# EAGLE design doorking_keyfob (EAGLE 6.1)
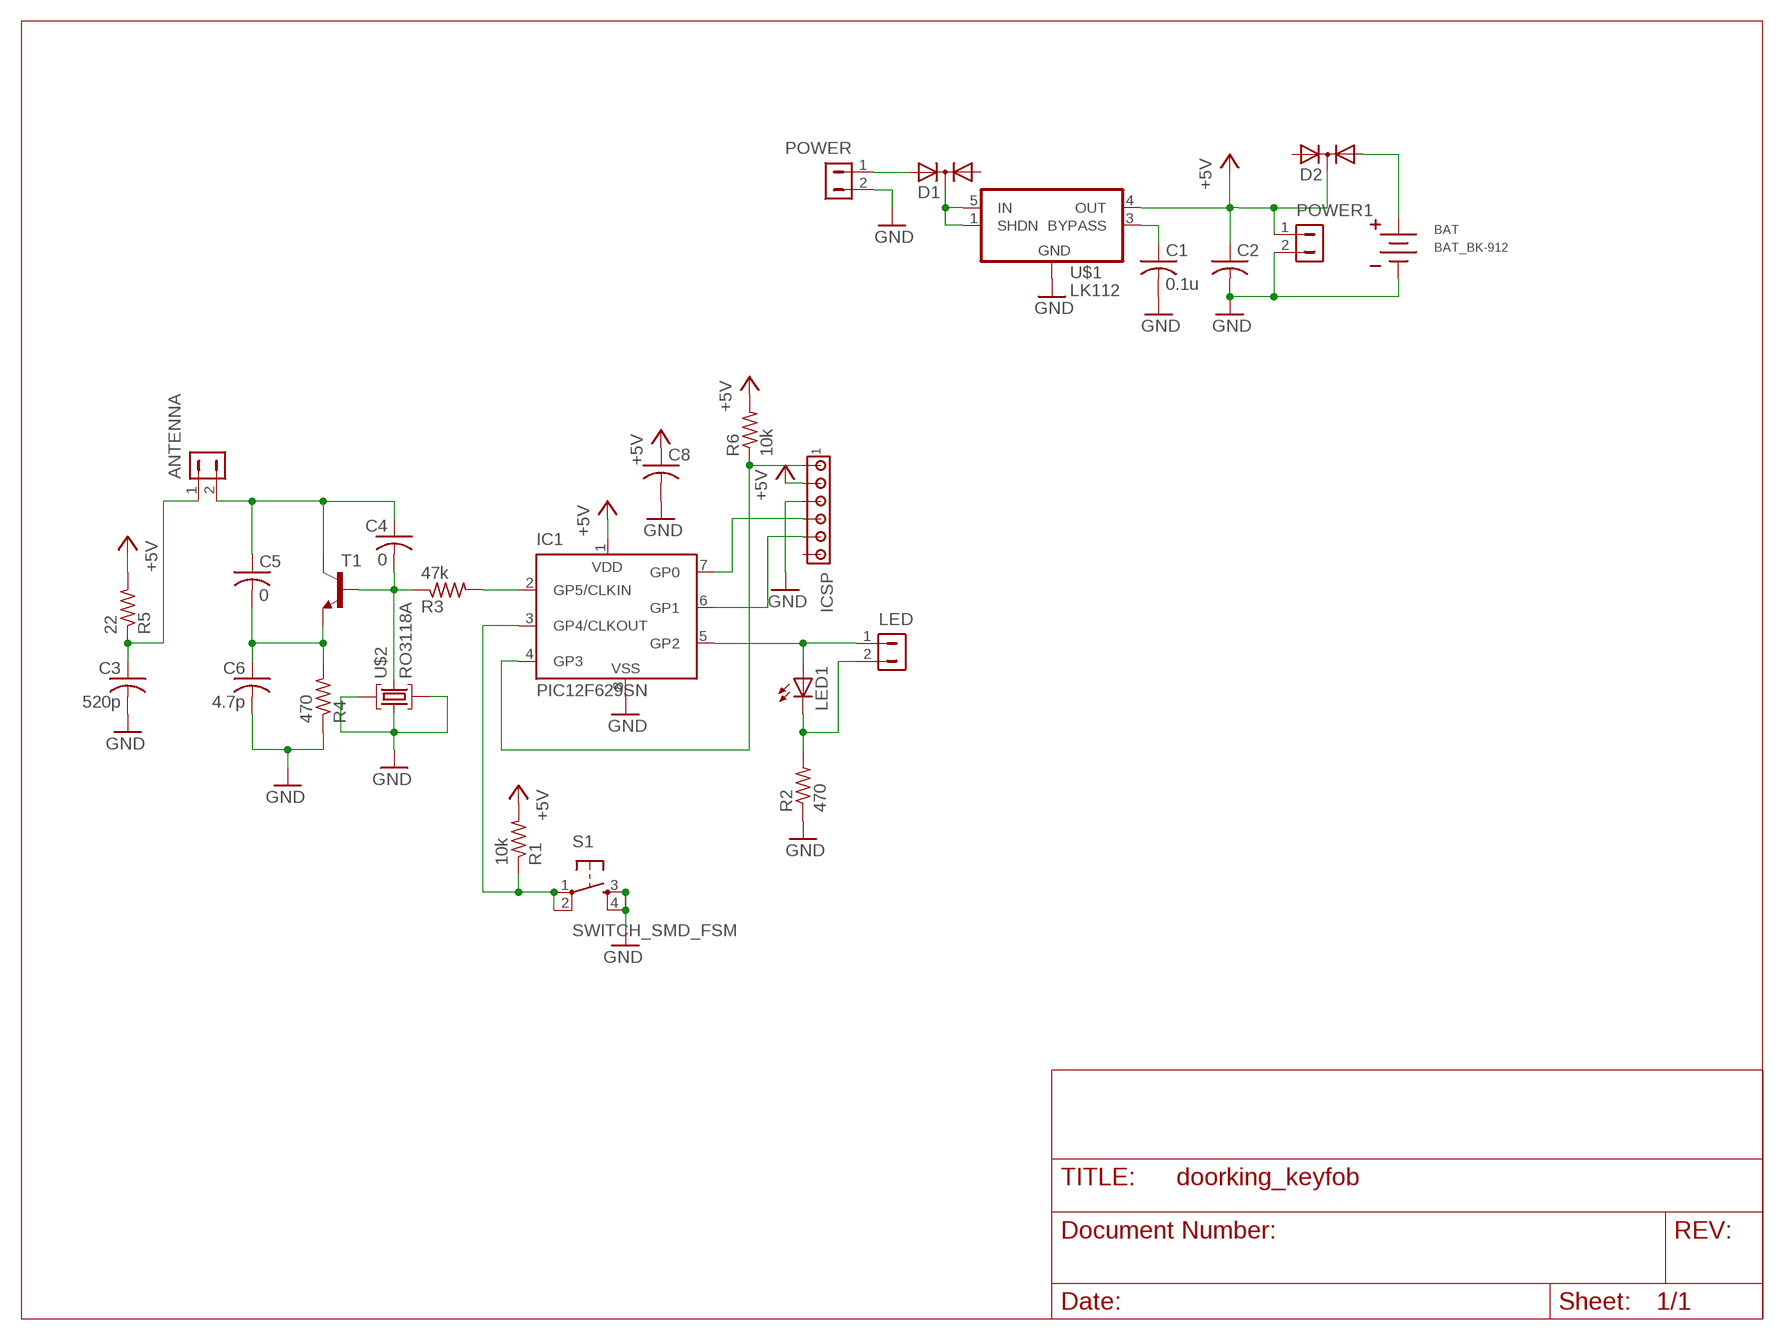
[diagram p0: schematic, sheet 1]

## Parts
ANTENNA  HDR-1X2-SIP-100  [SIP-100-2V]
BAT  BAT_BK-912  [BAT_BK-912]
C1  0.1u  C-USC0603  [C0603]
C2  C-USC0805  [C0805]
C3  520p  C-USC0603  [C0603]
C4  0  C-USC0603  [C0603]
C5  0  C-USC0603  [C0603]
C6  4.7p  C-USC0603  [C0603]
C8  C-USC0805  [C0805]
D1  DIODE-2AC|CASOT23  [SOT23]
D2  DIODE-2AC|CASOT23  [SOT23]
IC1  PIC12F629SN  [SO-08]
ICSP  MTA06-100  [10X06MTA]
LED  HDR-1X2-SIP-100  [SIP-100-2V]
LED1  LEDCHIPLED_1206  [CHIPLED_1206]
POWER  HDR-1X2-SIP-100  [SIP-100-2V]
POWER1  HDR-1X2-SIP-100  [SIP-100-2V]
R1  10k  R-US_R0603  [R0603]
R2  470  R-US_R0603  [R0603]
R3  47k  R-US_R0603  [R0603]
R4  470  R-US_R0603  [R0603]
R5  22  R-US_R0603  [R0603]
R6  10k  R-US_R0603  [R0603]
S1  SWITCH_SMD_FSM  [SWITCH_SMD_FSM]
T1  BFS17-NPN-SOT23-BEC  [SOT23-BEC]
U$1  LK112  [SOT23-5]
U$2  RO3118A  [RO3118A]

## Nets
+5V: C2.1 C8.1 D2.3(C) IC1.1(VDD) ICSP.5 POWER1.1 R1.2 R5.2 R6.2 U$1.4(OUT)
GND: BAT.NEG C1.2 C2.2 C3.2 C6.2 C8.2 IC1.8(VSS) ICSP.4 POWER1.2 POWER.2 R2.1 R4.1 S1.3 S1.4 U$1.2(GND) U$2.1 U$2.2 U$2.4
N$1: D1.3(C) U$1.1(SHDN) U$1.5(IN)
N$2: D1.2(A2) POWER.1
N$3: LED1.C LED.2 R2.2
N$4: IC1.3(GP4/CLKOUT) R1.1 S1.1 S1.2
N$5: IC1.5(GP2) LED1.A LED.1
N$6: IC1.2(GP5/CLKIN) R3.2
N$7: C4.2 R3.1 T1.B U$2.3
N$8: C1.1 U$1.3(BYPASS)
N$9: ANTENNA.2 C4.1 C5.1 T1.C
N$10: IC1.4(GP3) ICSP.6 R6.1
N$11: IC1.7(GP0) ICSP.3
N$12: IC1.6(GP1) ICSP.2
N$13: C5.2 C6.1 R4.2 T1.E
N$15: ANTENNA.1 C3.1 R5.1
VBAT: BAT.POS1(POS) BAT.POS2(POS) D2.1(A1)
Unconnected: D1.1(A1) D2.2(A2) ICSP.1

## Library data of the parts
ANTENNA LED POWER POWER1 = con-hdrs40:HDR-1X2: HEADER CONNECTOR
BAT = DSS:BAT_BK-912
C1-C6 C8 = rcl:C-US: CAPACITOR, American symbol
D1 D2 = diode:DIODE-2AC|CA: Dual DIODE Anode-Cathode|Cathode-Anode
IC1 = microchip:PIC12F6*: Data Sheet 8-Pin FLASH-Based 8-Bit CMOS Microcontrollers Source: http://www.microchip.com .. 41190c.pdf
ICSP = con-amp:MTA06-100: AMP connector
LED1 = led:LED: LED
R1-R6 = rcl:R-US_: RESISTOR, American symbol
S1 = DSS:SWITCH_SMD_FSM: SWITCH SMD TACTILE SPST-NO 0.05A 12V Digikey part 450-1759-1-ND
T1 = transistor:*-NPN-: NPN Transistror BF959 corrected 2008.03.06
U$1 = GT-IEEE:LK112
U$2 = GT-IEEE:RO3118A

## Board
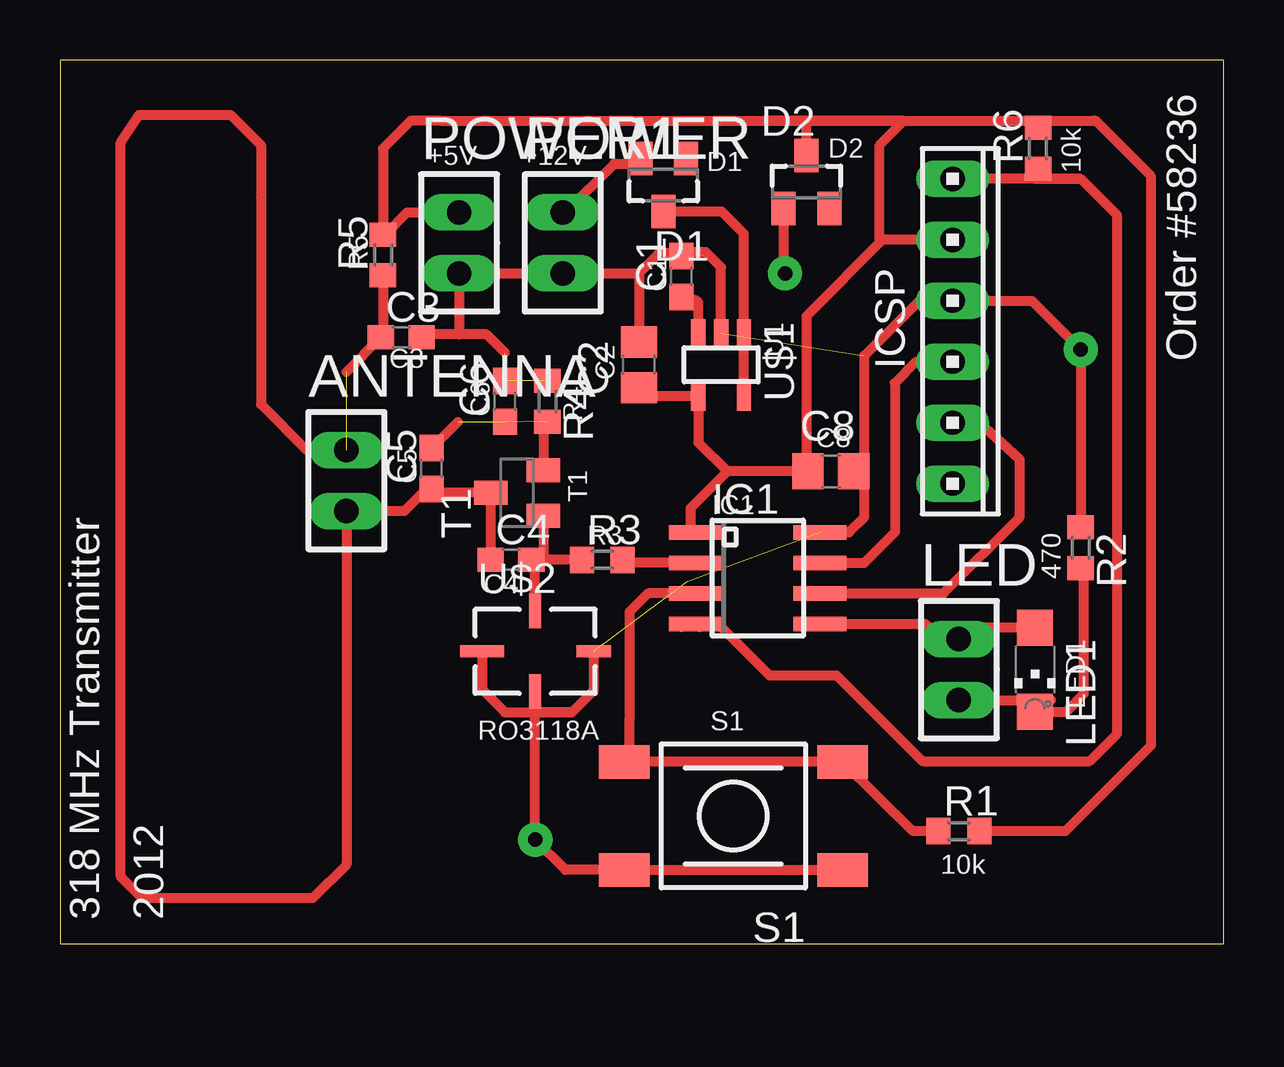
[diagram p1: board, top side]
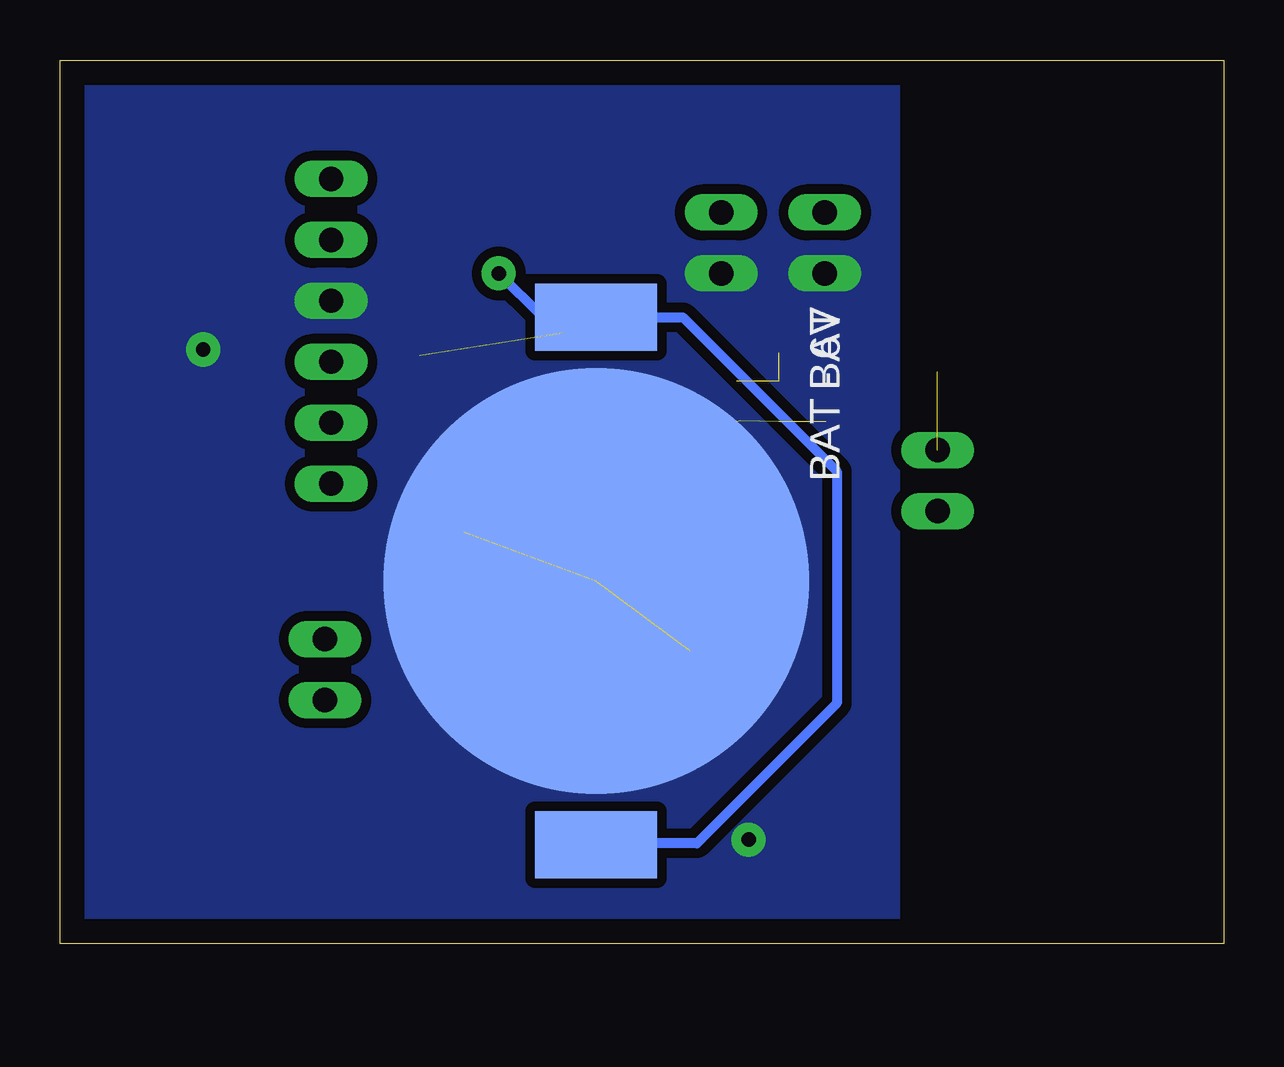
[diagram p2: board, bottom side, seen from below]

Size 48.51 x 36.83 mm. Coordinates in mm from the lower left corner, seen from the top.
Outline: 0,0 48.51,0 48.51,36.83 0,36.83 0,0
Copper layers (1*16): Top 0.035mm / dielectric 1.5mm / Bottom 0.035mm
Design rules: minimum track width 16mil, minimum drill 24mil, track to track 16mil, track to pad 16mil, pad to pad 16mil, via to via 16mil, smd to smd 16mil, copper to edge 40mil, drill to drill 8mil, minimum pad ring 10mil, minimum via ring 8mil, stop-mask expansion 4mil, vias tented up to drill 0mil, thermal gap 10mil

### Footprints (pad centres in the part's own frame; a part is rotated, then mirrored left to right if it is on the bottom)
SIP-100-2V = drill 1.016 long: 1 -1.27,0; 2 1.27,0
BAT_BK-912 = smd 17.74 x 17.74: NEG 0,0 | smd 2.79 x 5.08: POS1 10.99,0; POS2 -10.99,0
C0603 = smd 1.1 x 1: 1 -0.85,0; 2 0.85,0
C0805 = smd 1.3 x 1.5: 1 -0.95,0; 2 0.95,0
SOT23 = smd 1 x 1.4: 1 -0.95,-1.1; 2 0.95,-1.1; 3 0,1.1
SO-08 = smd 0.6 x 2.2: 1 -1.905,-2.6; 2 -0.635,-2.6; 3 0.635,-2.6; 4 1.905,-2.6; 5 1.905,2.6; 6 0.635,2.6; 7 -0.635,2.6; 8 -1.905,2.6
10X06MTA = drill 1.016 long: 1 6.35,0; 2 3.81,0; 3 1.27,0; 4 -1.27,0; 5 -3.81,0; 6 -6.35,0
CHIPLED_1206 = smd 1.5 x 1.5: A 0,-1.75; C 0,1.75
R0603 = smd 1 x 1.1: 1 -0.85,0; 2 0.85,0
SWITCH_SMD_FSM = smd 1.4 x 2.1: 1 2.25,4.55; 2 2.25,-4.55; 3 -2.25,4.55; 4 -2.25,-4.55
SOT23-BEC = smd 1 x 1.4: B -0.95,-1.1; C 0,1.1; E 0.95,-1.1
SOT23-5 = smd 0.6 x 1.2: 1 -0.95,-1.306; 2 0,-1.306; 3 0.95,-1.306; 4 0.95,1.306; 5 -0.95,1.306
RO3118A = smd 1.44 x 0.5: 1 1.68,0; 3 -1.68,0 | smd 0.5 x 1.84: 2 0,-2.22 | smd 0.5 x 1.44: 4 0,2.43

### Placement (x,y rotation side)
ANTENNA  11.94,19.3 270 top
BAT  26.16,15.11 270 bottom
C1  25.91,27.81 90 top
C2  24.13,24.13 90 top
C3  14.22,25.27 0 top
C4  18.8,16 0 top
C5  15.49,19.81 90 top
C6  18.54,22.61 90 top
C8  32.13,19.68 0 top
D1  25.15,31.62 180 top
D2  31.11,31.75 0 top
IC1  29.08,15.24 270 top
ICSP  37.21,25.53 270 top
LED  37.47,11.43 270 top
LED1  40.64,11.43 180 top
POWER  20.95,29.21 270 top
POWER1  16.64,29.21 270 top
R1  37.47,4.7 0 top
R2  42.55,16.51 270 top
R3  22.61,16 0 top
R4  20.32,22.61 270 top
R5  13.46,28.7 90 top
R6  40.77,33.15 90 top
S1  28.07,5.33 90 top
T1  19.05,18.8 90 top
U$1  27.56,24.13 180 top
U$2  19.81,12.19 270 top

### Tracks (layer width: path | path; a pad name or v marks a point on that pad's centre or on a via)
+5V
  Top 0.406: C2.1 24.36,22.82 U$1.4 26.61,20.89 27.81,19.68 | 29.34,34.29 29.21,34.29 15.88,34.29 14.61,34.29 13.46,33.15 R5.2 13.5,29.55 13.53,29.53 | 29.34,34.29 31.24,34.29 | 31.24,34.29 32.26,34.29 35.18,34.29 | R1.2 41.91,4.7 45.47,8.26 45.47,32 43.18,34.29 | 35.18,34.29 40.89,34.29 | 40.89,34.29 43.05,34.29 | 43.05,34.29 43.18,34.29 | 43.18,34.29 43.05,34.29 | 13.53,29.53 14.48,30.48 POWER1.1 | 13.53,29.53 13.46,29.46 | 27.81,19.68 C8.1 31.11,19.88 31.11,26.16 34.29,29.34 | 27.81,19.68 26.29,18.16 26.29,17.4 26.54,17.14 IC1.1 | ICSP.5 34.29,29.34 | 34.29,29.34 34.16,29.34 34.16,33.27 35.18,34.29 | R6.2 40.77,34.16 40.89,34.29 | 35.18,34.29 31.24,34.29 | 31.24,34.29 29.34,34.29 | D2.3 31.11,34.16 31.24,34.29
GND  (via drill 0.6 pad 1.42)  (5 unrouted)
  Top 0.406: 24.13,27.94 C2.2 | IC1.8 32.89,17.14 33.53,17.78 33.53,19.68 | POWER.2 21.08,27.94 | 21.08,27.94 24.13,27.94 | 33.53,19.68 C8.2 | R2.1 v42.55,24.77 40.51,26.8 ICSP.4 | U$2.4 22.24,10.56 21.34,9.65 | 21.34,9.65 19.84,9.65 | 19.84,9.65 19.81,9.65 | U$2.2 17.59,10.6 18.54,9.65 19.81,9.65 | 19.81,9.65 19.84,9.65 | 19.84,9.65 U$2.1 19.81,9.65 | 19.81,9.65 v19.81,4.34 21.07,3.08 S1.3 S1.4 | 19.81,9.65 19.84,9.65 | 19.84,9.65 21.34,9.65 | U$1.2 27.56,28.19 26.92,28.83 26.2,28.83 C1.2 | 24.13,27.94 24.98,28.79 25.82,28.79 25.91,28.7 C1.2 | 18.54,24.64 17.91,25.27 17.78,25.4 16.64,25.4 | 16.64,25.4 15.24,25.4 C3.2 | 21.08,27.94 POWER1.2 16.64,25.4 | 33.53,19.68 33.53,24.51 35.81,26.8 ICSP.4 | ICSP.4 37.34,26.8 ICSP.4 | C1.2 25.91,28.57 26.04,28.7 25.95,28.7 C1.2
  pour Bottom (no thermals): 13.72,0 48.39,-0.13 48.51,36.58 13.72,36.7
N$1
  Top 0.406: U$1.5 U$1.1 28.51,29.59 27.58,30.52 D1.3
N$2
  Top 0.406: POWER.1 21.08,30.48 23.11,32.51 24.13,32.51 | 24.13,32.51 24.26,32.51 | D1.2 24.17,32.47 24.13,32.51
N$3
  Top 0.406: LED.2 41.3,10.16 LED1.C 41.94,9.68 42.67,10.41 42.67,15.41 R2.2
N$4
  Top 0.406: R1.1 35.56,4.7 S1.2 S1.1 23.52,7.77 23.75,8 23.75,9.4 23.75,13.84 24.51,14.61 IC1.3
N$5
  Top 0.406: IC1.5 36.07,13.34 36.7,12.7 LED.1 37.82,13.18 LED1.A
N$6
  Top 0.406: IC1.2 23.58,15.88 R3.2
N$7
  Top 0.406: R3.1 20.32,16 | 20.32,16 C4.2 19.81,15.84 19.81,15.75 U$2.3 | T1.B 20.15,16.17 20.32,16
N$8
  Top 0.406: U$1.3 26.61,26.73 26.54,26.8 C1.1
N$9
  Top 0.406: C4.1 T1.C 15.66,18.8 C5.1 15.28,18.96 14.35,18.03 12.06,18.03 | 12.06,18.03 ANTENNA.2 | 12.06,18.03 11.94,17.91 11.94,3.3 10.54,1.91 3.43,1.91 2.54,2.79 2.54,33.4 3.3,34.54 7.11,34.54 8.38,33.27 8.38,31.11 8.38,22.48 10.29,20.57 12.06,20.57
N$10
  Top 0.406: 42.55,31.88 44.07,30.35 44.07,8.76 42.93,7.62 35.94,7.62 32.38,11.18 30.86,11.18 29.59,11.18 27.56,13.21 26.67,13.21 | 42.55,31.88 40.64,31.88 | 40.64,31.88 ICSP.6 | 26.67,13.21 25.91,13.21 25.78,13.34 IC1.4 | IC1.4 26.54,13.34 | 26.54,13.34 26.67,13.21 | 26.67,13.21 26.54,13.34 | 26.54,13.34 IC1.4 | R6.1 40.77,32 40.64,31.88 | 40.64,31.88 42.55,31.88
N$11
  Top 0.406: IC1.7 33.53,15.88 34.8,17.14 34.8,23.37 35.69,24.26 ICSP.3
N$12
  Top 0.406: IC1.6 34.16,14.61 36.83,14.61 40.01,17.78 40.01,20.19 38.35,21.72 ICSP.2
N$13  (3 unrouted)
  Top 0.406: T1.E 20.15,21.8 20.32,21.97 | 16.59,21.76 C5.2
N$15  (1 unrouted)
  Top 0.406: 11.94,23.84 C3.1 13.46,25.44 R5.1
VBAT  (via drill 0.6 pad 1.42)
  Top 0.406: D2.1 30.16,28 v30.23,27.94
  Bottom 0.406: v30.23,27.94 28.39,26.1 BAT.POS2 22.55,26.1 16.13,19.68 16.13,10.03 21.97,4.19 26.09,4.19 BAT.POS1

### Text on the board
_tsilk: Order #58236 | +5V | +12V | D1 | D2 | 10k | R5 | ICSP | C1 | U1 | C3 | R4 | C2 | C6 | C8 | C5 | T1 | IC1 | R3 | 470 | C4 | LED1 | S1 | RO3118A | 10k | 318 MHz Transmitter | 2012
_bsilk: BAT - 6V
